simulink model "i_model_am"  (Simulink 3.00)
settings: Solver=ode45  StartTime=0.0  StopTime=10.0  RelTol=1e-3
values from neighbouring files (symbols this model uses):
  J = 0.0017    [Data.m]
  kr = Lm/Lr    (= 0.963591022444)    [Data.m]
  Lm = .5796    (= 0.5796)    [Data.m]
  p = 1    [Data.m]
  Tr = Lr/Rr    (= 0.162567567568)    [Data.m]

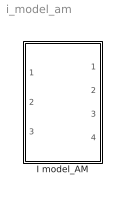
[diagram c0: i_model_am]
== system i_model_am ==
  I model_AM : Subsystem

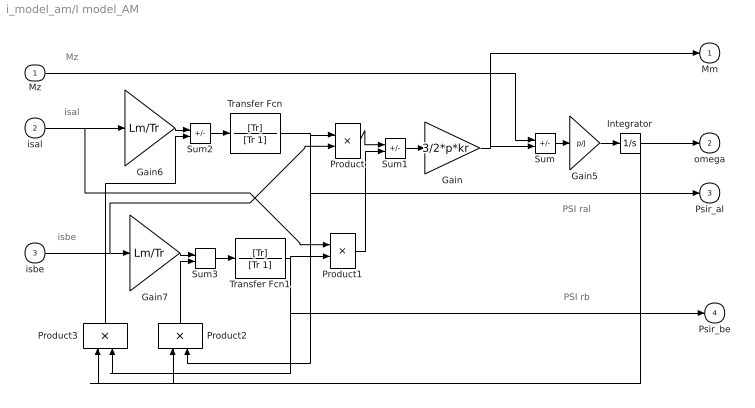
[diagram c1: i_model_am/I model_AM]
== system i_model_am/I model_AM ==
  note: isal
  note: PSI ral
  note: isbe
  note: PSI rb
  note: Mz
  Mz : Inport  Port=1  PortWidth=-1  SampleTime=-1  DataType=auto
  isal : Inport  Port=2  PortWidth=-1  SampleTime=-1  DataType=auto
  isbe : Inport  Port=3  PortWidth=-1  SampleTime=-1  DataType=auto
  Gain : Gain  Gain=3/2*p*kr  SaturateOnIntegerOverflow=on
  Gain5 : Gain  Gain=p/J  SaturateOnIntegerOverflow=on
  Gain6 : Gain  Gain=Lm/Tr  SaturateOnIntegerOverflow=on
  Gain7 : Gain  Gain=Lm/Tr  SaturateOnIntegerOverflow=on
  Integrator : Integrator  ExternalReset=none  InitialConditionSource=internal  InitialCondition=0  LimitOutput=off  UpperSaturationLimit=inf  LowerSaturationLimit=-inf  ShowSaturationPort=off  ShowStatePort=off  AbsoluteTolerance=auto
  Product : Product  Inputs=2  SaturateOnIntegerOverflow=on
  Product1 : Product  Inputs=2  SaturateOnIntegerOverflow=on
  Product2 : Product  Orientation=up  Inputs=2  SaturateOnIntegerOverflow=on
  Product3 : Product  Orientation=up  Inputs=2  SaturateOnIntegerOverflow=on
  Sum : Sum  Inputs=-+  SaturateOnIntegerOverflow=on
  Sum1 : Sum  Inputs=+-  SaturateOnIntegerOverflow=on
  Sum2 : Sum  Inputs=+-  SaturateOnIntegerOverflow=on
  Sum3 : Sum  Inputs=++  SaturateOnIntegerOverflow=on
  Transfer Fcn : TransferFcn  Numerator=[Tr]  Denominator=[Tr 1]
  Transfer Fcn1 : TransferFcn  Numerator=[Tr]  Denominator=[Tr 1]
  Mm : Outport  Port=1  InitialOutput=0
  omega : Outport  Port=2  InitialOutput=0
  Psir_al : Outport  Port=3  InitialOutput=0
  Psir_be : Outport  Port=4  InitialOutput=0
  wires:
  Gain/1 -> Mm/1, Sum/2
  Product1/1 -> Sum1/2
  Mz/1 -> Sum/1
  isbe/1 -> Gain7/1, Product/2
  Product2/1 -> Sum3/2
  Sum3/1 -> Transfer Fcn1/1
  Sum2/1 -> Transfer Fcn/1
  Product/1 -> Sum1/1
  Sum1/1 -> Gain/1
  Sum/1 -> Gain5/1
  Integrator/1 -> omega/1, Product3/1, Product2/1
  Transfer Fcn/1 -> Product/1, Product2/2, Psir_al/1
  Gain7/1 -> Sum3/1
  Gain6/1 -> Sum2/1
  Transfer Fcn1/1 -> Product1/2, Product3/2, Psir_be/1
  Product3/1 -> Sum2/2
  isal/1 -> Gain6/1, Product1/1
  Gain5/1 -> Integrator/1
